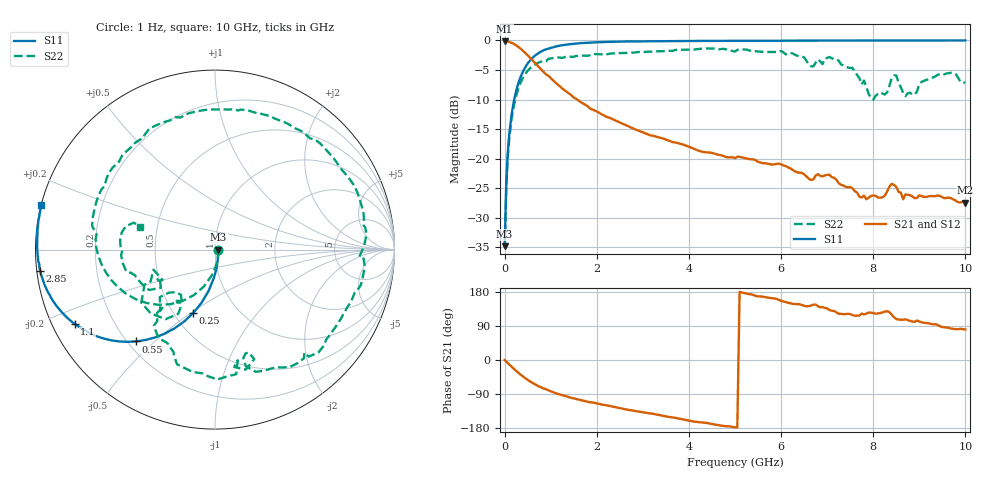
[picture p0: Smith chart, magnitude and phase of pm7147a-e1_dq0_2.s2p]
# GHz S DB R 50
! S-Parameters data
! Freq  dbS11  angS11  dbS21  angS21  dbS12  angS12  dbS22  angS22
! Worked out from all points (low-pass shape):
!   279 points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, 1 Hz to 10 GHz, reference 50 ohm
!   highest |S21| = -0.16 dB at 3.981 kHz (marker M1); lowest = -27.4 dB at 10 GHz (marker M2)
!   |S21| within 3 dB of the highest: start of sweep to 580 MHz
!   lowest |S11| = -34.8 dB at 3.981 kHz (marker M3), VSWR 1.04, Z = 51.9 - j0.000591 ohm
!   |S11| at or under -10 dB: start of sweep to 208.2 MHz
!   |S22| runs from -34.8 to -1.4 dB; largest |S21 - S12| = 1.4e-12
!   S11 on the Smith chart (normalised r, x): 1 Hz: 1.04, -0.00; 250 MHz: 0.62, -0.51; 550 MHz: 0.23, -0.44; 1.1 GHz: 0.06, -0.25; 2.85 GHz: 0.01, -0.06; 10 GHz: 0.00, +0.13
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1e-09  -34.79 -0.0  -0.16 -0.0  -0.16 -0.0  -34.79 -0.0
3.9811e-06  -34.79 -0.0  -0.16 -0.0  -0.16 -0.0  -34.79 -0.0
0.03981072  -23.60 -77.3  -0.18 -4.7  -0.18 -4.7  -24.28 -78.2
0.07943282  -17.92 -88.9  -0.23 -9.4  -0.23 -9.4  -18.63 -92.6
0.25  -8.55 -108.9  -0.84 -28.7  -0.84 -28.7  -9.40 -122.3
0.55  -3.42 -130.7  -2.92 -56.4  -2.92 -56.4  -4.73 -158.9
1.1  -1.06 -152.2  -7.11 -87.1  -7.11 -87.1  -2.95 158.4
1.7  -0.45 -163.1  -10.65 -106.9  -10.65 -106.9  -2.58 127.1
2.85  -0.16 -173.1  -15.10 -135.0  -15.10 -135.0  -2.01 79.5
3.35  -0.14 -175.7  -16.41 -145.0  -16.41 -145.0  -1.83 60.0
4.35  -0.09 -179.9  -18.91 -165.4  -18.91 -165.4  -1.36 22.2
5.05  -0.08 177.8  -19.67 -177.8  -19.67 -177.8  -1.62 -3.5
6.05  -0.06 175.0  -21.15 154.5  -21.15 154.5  -2.02 -48.8
6.7  -0.04 173.2  -23.49 146.2  -23.49 146.2  -4.39 -71.9
7.05  -0.04 172.4  -22.72 131.9  -22.72 131.9  -2.81 -89.0
7.6  -0.03 171.1  -25.50 116.8  -25.50 116.8  -5.28 -128.8
8  -0.03 170.1  -26.21 123.9  -26.21 123.9  -10.04 -127.0
8.35  -0.04 169.3  -24.73 126.3  -24.73 126.3  -7.70 -119.7
8.5  -0.03 169.0  -24.77 108.1  -24.77 108.1  -5.93 -144.3
8.7  -0.03 168.6  -26.03 107.4  -26.03 107.4  -9.43 -149.9
9.5  -0.02 166.8  -26.52 86.9  -26.52 86.9  -5.61 -176.6
10  -0.02 165.7  -27.42 80.6  -27.42 80.6  -7.18 163.5
